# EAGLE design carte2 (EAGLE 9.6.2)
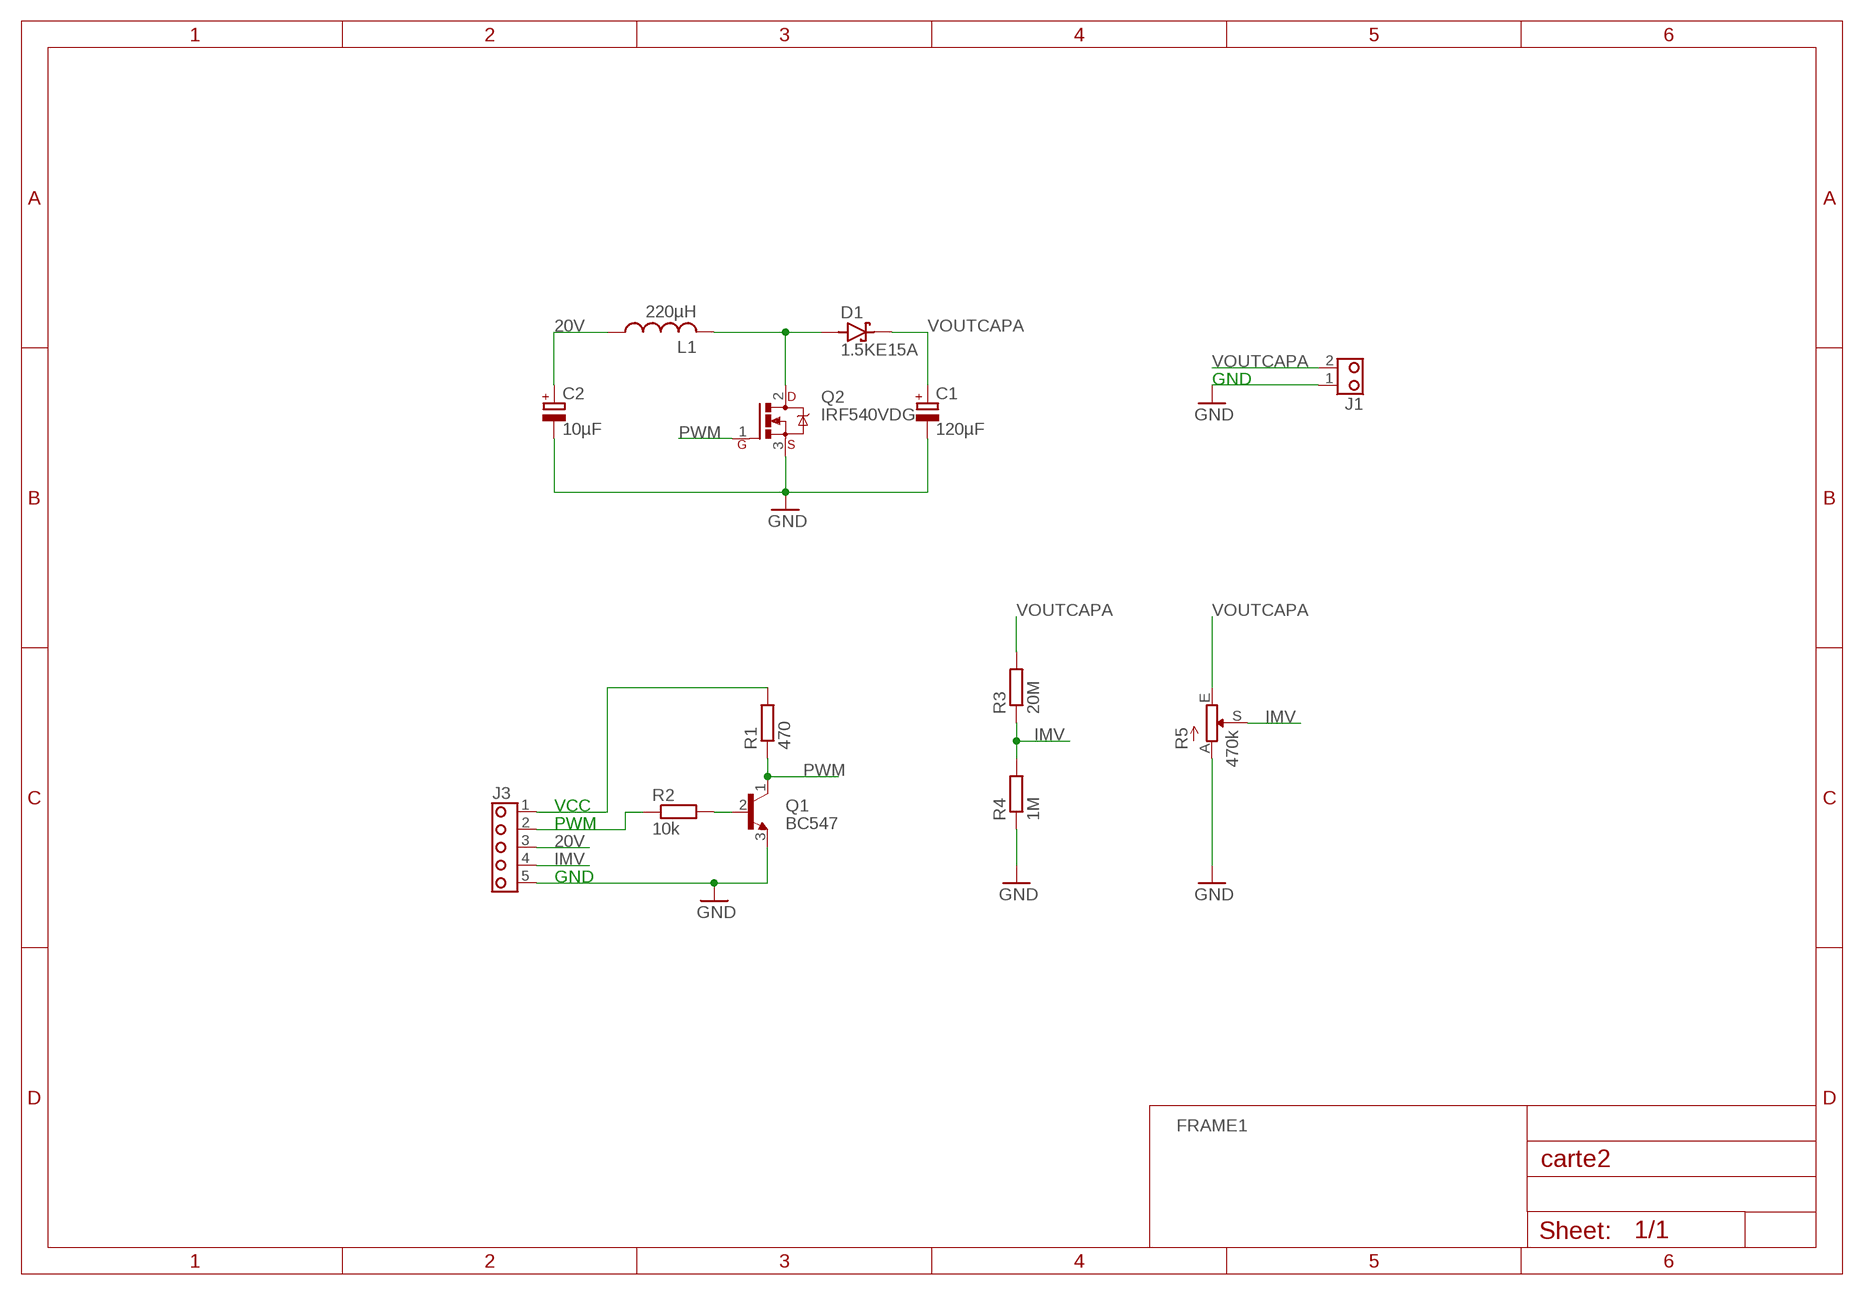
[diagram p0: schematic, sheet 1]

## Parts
C1  120µF  C_POL-E2,5-7  [E2,5-7]
C2  10µF  C_POL-E2,5-7  [E2,5-7]
D1  1.5KE15A  [DO-201AD-15]
J1  BORNIER_2-D2P  [MSTBA2]
J3  BORNIER_5-D5P  [MSTBA5]
L1  220µH  L-1400  [1422455C]
Q1  BC547  [TO92]
Q2  IRF540VDG  [TO220VDG]
R1  470  R-0207/12  [R0207/12]
R2  10k  R-0207/12  [R0207/12]
R3  20M  R-0207/12  [R0207/12]
R4  1M  R-0207/12  [R0207/12]
R5  470k  POTT93YA  [T93YA]

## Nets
20V: C2.+ J3.3 L1.1
GND: C1.- C2.- J1.1 J3.5 Q1.3(E) Q2.3(S) R4.1 R5.A
IMV: J3.4 R3.1 R4.2 R5.S
N$2: J3.2 R2.1
N$4: Q1.2(B) R2.2
N$8: D1.A L1.2 Q2.2(D)
N$11: J3.1 R1.2
PWM: Q1.1(C) Q2.1(G) R1.1
VOUTCAPA: C1.+ D1.C J1.2 R3.2 R5.E

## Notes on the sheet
- GND
- VCC
- PWM
- GND

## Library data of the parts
C1 C2 = 0IUT RLCQ:C_POL: Condensateur Polarisé; MAGASIN: (Armoire n°1)
D1 = 0IUT DT:1.5KE15A: DIODE Transil Unidirectionnelle 1500W; MAGASIN: TRANSIL (Tiroirs n°4-6)
J1 = 0IUT CONNECTEURS:BORNIER_2: BORNIER, 2 Contacts; MAGASIN: Bornier D2P (Armoire n°4) Bornier D2PF (Armoire n°4)
J3 = 0IUT CONNECTEURS:BORNIER_5: BORNIER, 5 Contacts GEII/IUT ANGERS; MAGASIN: Bornier D5P (Armoire n°4) Bornier D5PF (Armoire n°4)
L1 = 0IUT RLCQ:L: INDUCTANCE, Symbole Américain; MAGASIN: SELF (Tiroirs n°3-3)
Q1 = 0IUT DT:BC547: Transistor NPN Amplificateur Vceo: 45V Ic: 100mA Doc constructeur Détails/équivalence: http://geii/composants/ GEII/IUT ANGERS; MAGASIN: Transistors (Tiroirs n°4-1)
Q2 = 0IUT DT:IRF540: Transistor MOSFET CANAL N de Puissance (Low Gate Charge) Vds: 100V Id: 22A P: 85W Doc constructeur Détails/équivalence: http://geii/composants/ GEII/IUT ANGERS; MAGASIN: FET-MOSFET (Tiroirs n°4-3) Dissipateur-G (Armoire n°5)
R1-R4 = 0IUT RLCQ:R: Résistance Européenne; MAGASIN: (Armoire n°2)
R5 = 0IUT RLCQ:POT: POTENTIOMETRE Voir les valeurs sur site Magasin: http://geii/magasin GEII/IUT ANGERS; MAGASIN: (Armoire n°6)

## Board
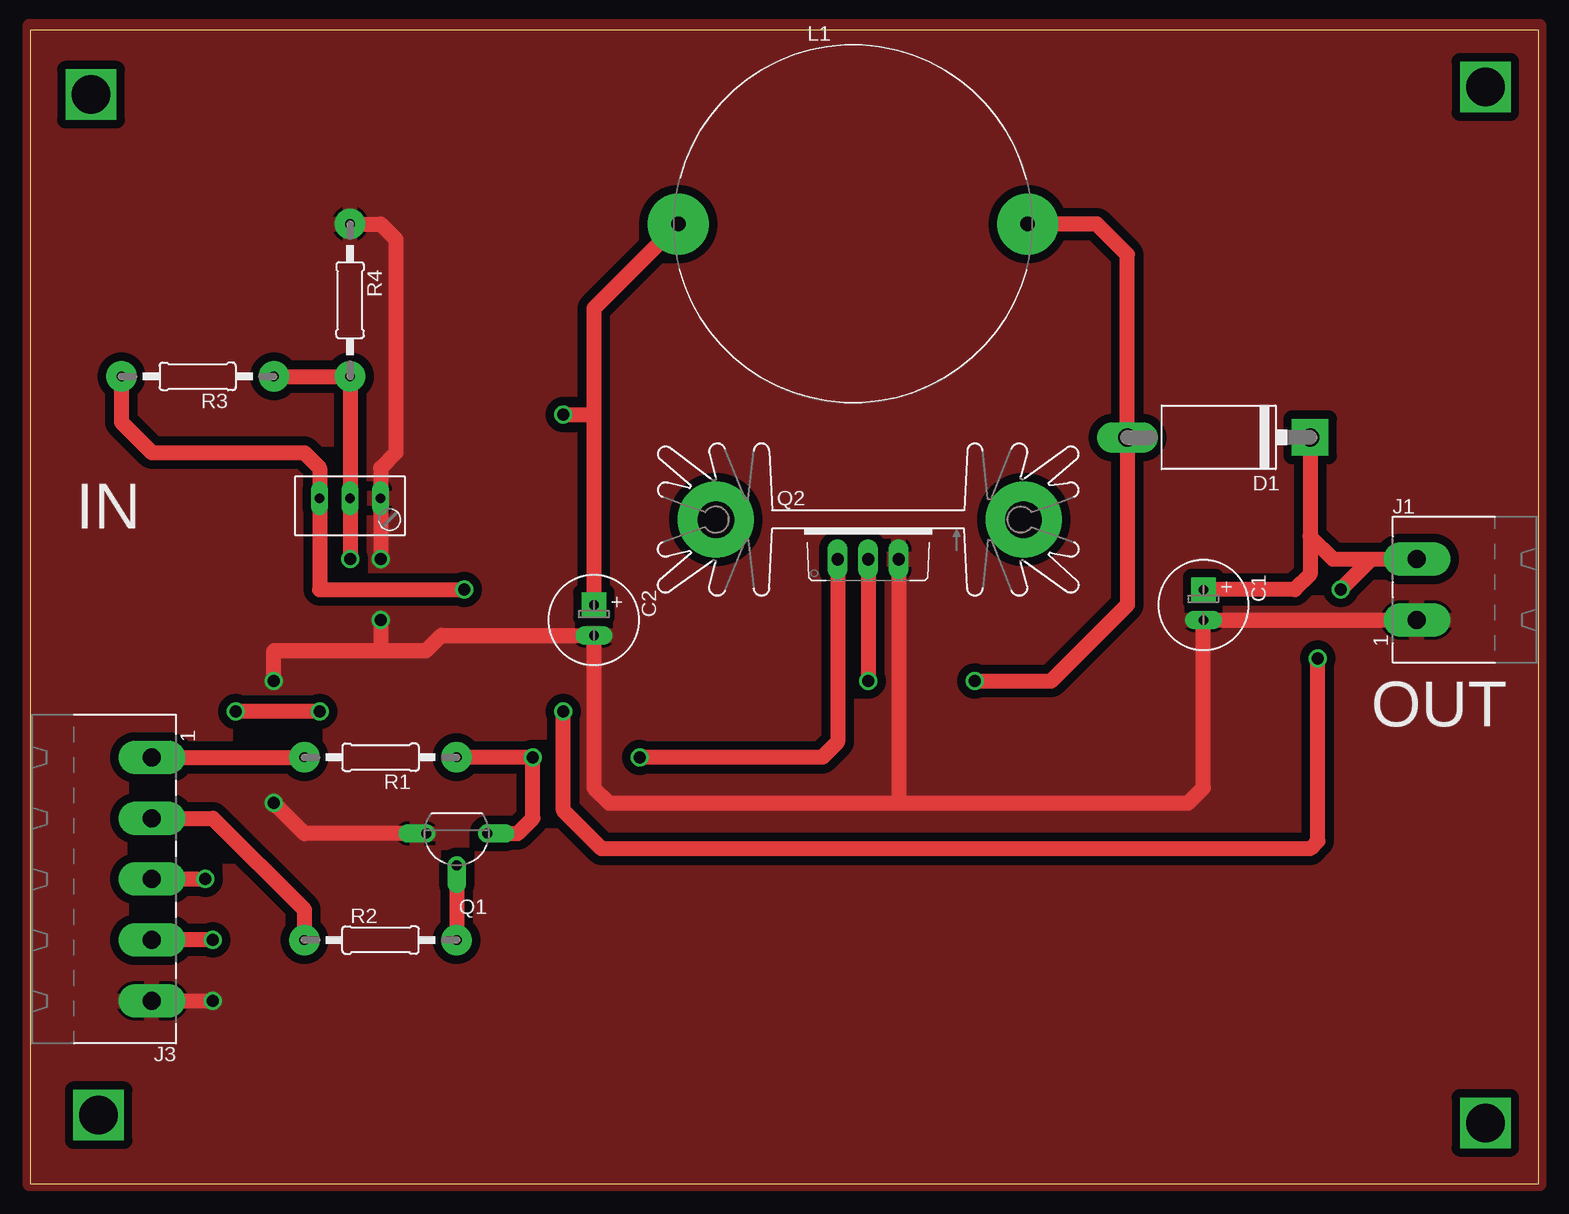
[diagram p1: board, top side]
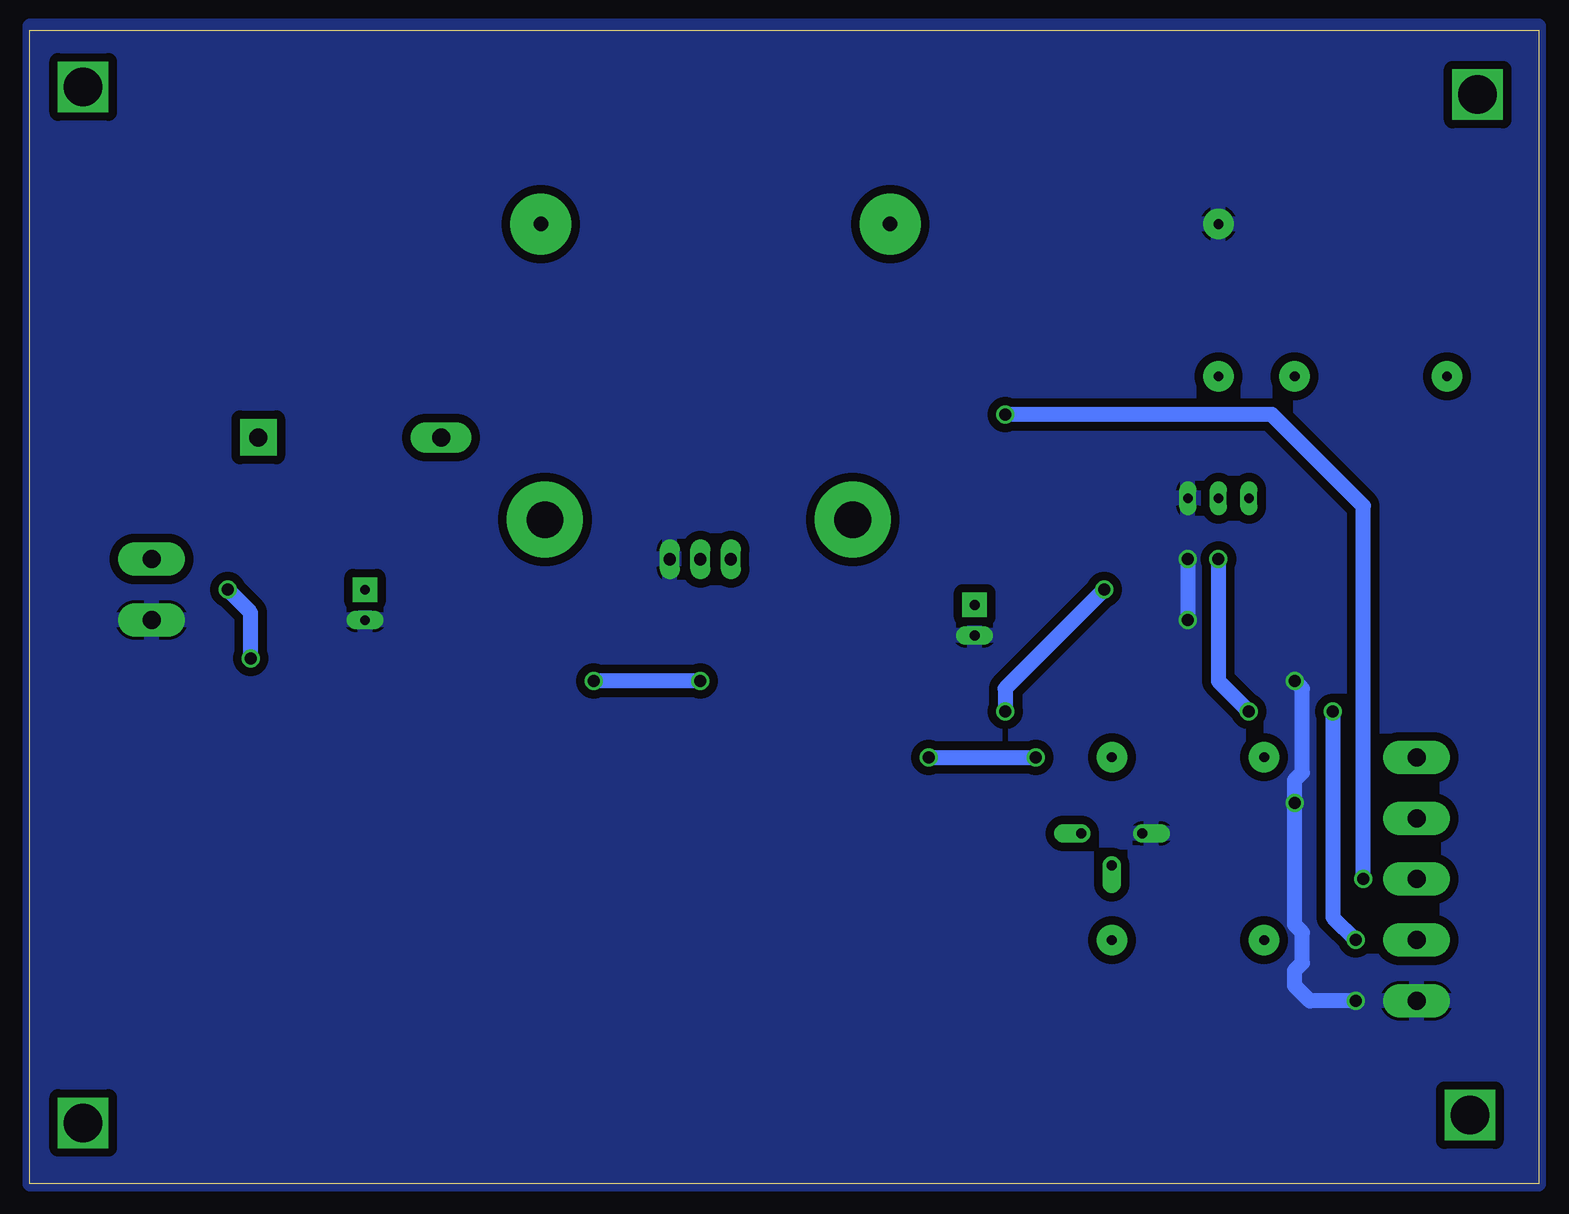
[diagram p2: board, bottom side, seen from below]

Size 125.71 x 96.19 mm. Coordinates in mm from the lower left corner, seen from the top.
Outline: 0,0 125.71,0 125.71,96.19 0,96.19 0,0
Copper layers (1*16): Top 0.035mm / dielectric 1.5mm / Bottom 0.035mm
Design rules "default *": minimum track width 6mil, minimum drill 0.35mm, track to track 28mil, track to pad 28mil, pad to pad 6mil, via to via 6mil, smd to smd 6mil, copper to edge 0mil, drill to drill 30mil, minimum pad ring 10mil, minimum via ring 8mil, stop-mask expansion 4mil, vias tented up to drill 0mil, thermal gap 10mil

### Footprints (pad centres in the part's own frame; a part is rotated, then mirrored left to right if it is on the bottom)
E2,5-7 = drill 0.813 pad 2.032 square: + -1.27,0 | drill 0.813 pad 1.524 long: - 1.27,0
DO-201AD-15 = drill 1.499 pad 2.54 long: A 7.62,0 | drill 1.499 pad 3.048 square: C -7.62,0
MSTBA2 = drill 1.499 pad 2.794 long: 1 -2.54,0; 2 2.54,0
MSTBA5 = drill 1.499 pad 2.794 long: 1 -10.16,0; 2 -5.08,0; 3 0,0; 4 5.08,0; 5 10.16,0
1422455C = drill 1.219 pad 5.08: 1 -14.55,0; 2 14.55,0
TO92 = drill 0.813 pad 1.524 offset: 1 -2.54,0; 2 0,2.667; 3 2.54,0
TO220VDG = drill 1.016 pad 1.676 long: 1 -2.54,-2.54; 2 0,-2.54; 3 2.54,-2.54 | drill 3.048 pad 6.35: K1 12.954,0.762; K2 -12.7,0.762
R0207/12 = drill 0.813 pad 2.54: 1 -6.35,0; 2 6.35,0
T93YA = drill 0.813 pad 1.422 long: A 2.54,0; E -2.54,0; S 0,0

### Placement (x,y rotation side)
C1  97.79,48.26 270 top
C2  46.99,46.99 270 top
D1  99.06,62.23 180 top
J1  115.57,49.53 90 top
J3  10.16,25.4 270 top
L1  68.58,80.01 0 top
Q1  35.56,29.21 180 top
Q2  69.85,54.61 0 top
R1  29.21,35.56 180 top
R2  29.21,20.32 0 top
R3  13.97,67.31 180 top
R4  26.67,73.66 270 top
R5  26.67,57.15 0 top

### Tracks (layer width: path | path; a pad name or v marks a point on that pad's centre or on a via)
20V  (via drill 1)
  Top 1.27: L1.1 46.99,72.97 46.99,64.14 | 46.99,64.14 C2.+ | J3.3 v14.61,25.4 | v44.45,64.14 46.99,64.14
  Bottom 1.27: v14.61,25.4 14.61,56.52 22.23,64.14 v44.45,64.14
GND  (via drill 1)
  Top 1.27: 29.21,44.45 20.32,44.45 v20.32,41.91 | Q2.3 72.39,31.75 | 72.39,31.75 96.52,31.75 97.79,33.02 C1.- J1.1 | 29.21,44.45 33.02,44.45 34.29,45.72 C2.- 46.99,33.02 48.26,31.75 72.39,31.75 | R4.1 29.21,80.01 30.48,78.74 30.48,60.96 29.21,59.69 R5.A v29.21,52.07 | v29.21,46.99 29.21,44.45 | Q1.3 22.86,29.21 v20.32,31.75 | J3.5 v15.24,15.24
  Bottom 1.27: v29.21,52.07 v29.21,46.99 | v15.24,15.24 19.05,15.24 20.32,16.51 20.32,17.78 19.68,18.41 19.68,20.95 20.32,21.59 v20.32,31.75 20.32,33.66 19.68,34.29 19.68,41.27 v20.32,41.91
  pour Bottom: 0,96.52 125.73,96.52 125.73,0 0,0
  pour Top: 0,96.52 125.73,96.52 125.73,0 0,0
IMV  (via drill 1)
  Top 1.27: R3.1 R4.2 R5.S v26.67,52.07 | v24.13,39.37 v17.14,39.37 | v15.24,20.32 J3.4
  Bottom 1.27: v26.67,52.07 26.67,41.91 v24.13,39.37 | v17.14,39.37 17.14,22.23 v15.24,20.32
N$1  (via drill 3.2)
  other vias: 5.71,5.71
N$2
  Top 1.27: J3.2 15.24,30.48 22.86,22.86 R2.1
N$3  (via drill 3.2)
  other vias: 5.08,90.8
N$4
  Top 1.27: Q1.2 R2.2
N$5  (via drill 3.2)
  other vias: 121.28,91.44
N$7  (via drill 3.2)
  other vias: 121.28,5.08
N$8  (via drill 1)
  Top 1.27: Q2.2 v69.85,41.91 | v78.74,41.91 85.09,41.91 91.44,48.26 D1.A 91.44,77.47 88.9,80.01 L1.2
  Bottom 1.27: v69.85,41.91 v78.74,41.91
N$11
  Top 1.27: J3.1 R1.2
PWM  (via drill 1)
  Top 1.27: v50.8,35.56 66.04,35.56 67.31,36.83 Q2.1 | R1.1 v41.91,35.56 41.91,30.48 40.64,29.21 Q1.1
  Bottom 1.27: v50.8,35.56 v41.91,35.56
VOUTCAPA  (via drill 1)
  Top 1.27: C1.+ 105.41,49.53 106.68,50.8 D1.C 106.68,53.97 108.58,52.07 J1.2 111.76,52.07 v109.22,49.53 | R3.2 7.62,63.5 10.16,60.96 22.86,60.96 24.13,59.69 R5.E 24.13,49.53 v36.2,49.53 | v44.45,39.37 44.45,31.11 47.62,27.94 106.68,27.94 107.31,28.57 v107.31,43.81
  Bottom 1.27: v36.2,49.53 44.45,41.27 v44.45,39.37 | v107.31,43.81 107.31,47.62 v109.22,49.53

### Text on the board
tNames: IN | OUT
